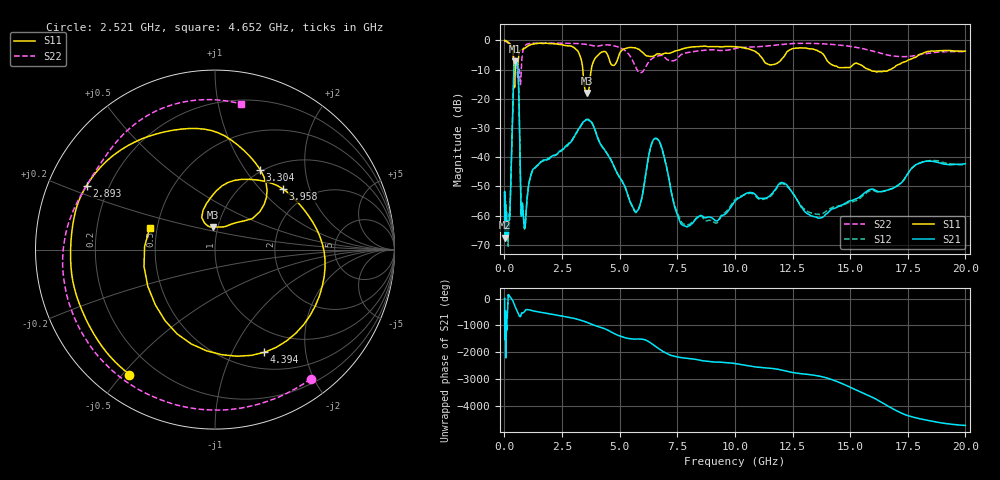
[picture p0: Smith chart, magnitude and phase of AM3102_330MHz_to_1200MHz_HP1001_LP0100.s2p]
! Date/Time: Tue, Sep 11, 2018 5:18 PM
! Network Analyzer: Agilent Technologies E8362B Rev: A.07.50.63
! Sweep from 0.010 to 20.000 GHz, 1601 Points, Sweep Type: LOG
! Power Supply: 4.949 V, 0.001 A
# Hz S DB R 50
!freq MagS11 AngS11 MagS21 AngS21 MagS12 AngS12 MagS22 AngS22
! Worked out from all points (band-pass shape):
!   1601 points, 10 MHz to 20 GHz, reference 50 ohm
!   highest |S21| = -7.09 dB at 464.5 MHz (marker M1); lowest = -67.6 dB at 42.99 MHz (marker M2)
!   |S21| within 3 dB of the highest: 415.1 MHz to 590.3 MHz (175.3 MHz wide, 34.9 % of centre)
!   lowest |S11| = -18.0 dB at 3.599 GHz (marker M3), VSWR 1.29, Z = 47.6 + j12.1 ohm
!   |S11| at or under -10 dB: 418.3 MHz to 469.3 MHz (51.07 MHz wide, 11.5 % of centre); 3.403 GHz to 3.769 GHz (365.6 MHz wide, 10.2 % of centre); 15.84 GHz to 16.72 GHz (881.5 MHz wide, 5.41 % of centre)
!   |S22| runs from -15.1 to -0.2 dB; largest |S21 - S12| = 0.0059
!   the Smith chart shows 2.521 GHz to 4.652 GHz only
!   S11 on the Smith chart (normalised r, x): 2.521 GHz: 0.11, -0.52; 2.893 GHz: 0.12, +0.23; 3.304 GHz: 0.97, +1.17; 3.958 GHz: 1.48, +1.35; 4.394 GHz: 0.70, -1.34; 4.652 GHz: 0.46, +0.13
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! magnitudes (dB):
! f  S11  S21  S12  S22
! 10 MHz  0.0  -61.1  -53.7  -0.2
! 35.55 MHz  0.0  -63.0  -65.5  -0.3
! 42.99 MHz  0.0  -67.6  -65.8  -0.3
! 126.4 MHz  -0.4  -64.3  -64.0  -0.7
! 226.7 MHz  -1.1  -59.3  -61.5  -1.3
! 447.2 MHz  -15.9  -7.3  -7.3  -6.9
! 464.5 MHz  -11.3  -7.1  -7.2  -6.5
! 591.9 MHz  -7.7  -10.3  -10.4  -13.0
! 722.6 MHz  -3.2  -58.9  -58.6  -12.4
! 869.7 MHz  -2.7  -64.1  -64.3  -2.0
! 1.59 GHz  -1.0  -41.6  -41.6  -0.9
! 2.521 GHz  -1.5  -37.3  -37.5  -1.0
! 2.893 GHz  -1.9  -34.7  -34.5  -1.0
! 3.304 GHz  -5.8  -29.4  -29.4  -1.1
! 3.599 GHz  -18.0  -27.2  -27.0  -1.4
! 3.958 GHz  -5.9  -31.4  -31.3  -2.0
! 4.394 GHz  -3.9  -38.1  -38.0  -1.5
! 4.652 GHz  -8.3  -41.4  -41.5  -1.7
! 5.652 GHz  -2.5  -58.4  -58.6  -8.4
! 6.549 GHz  -5.0  -33.5  -33.7  -5.6
! 7.882 GHz  -2.6  -63.8  -63.1  -4.3
! 20 GHz  -3.7  -42.3  -42.7  -3.8
